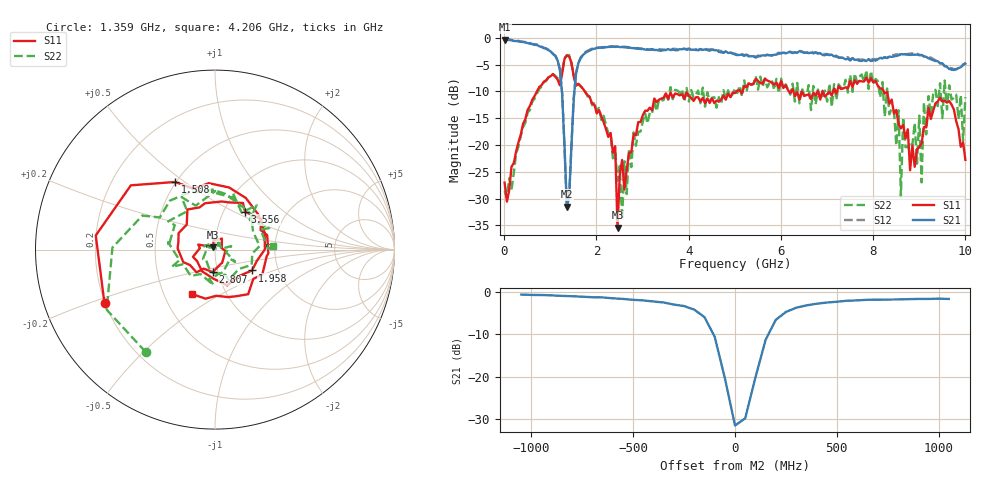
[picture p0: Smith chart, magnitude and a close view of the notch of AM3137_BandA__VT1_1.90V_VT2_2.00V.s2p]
! Date/Time: Tue, Nov 13, 2018 4:48 PM
! Network Analyzer: Agilent Technologies E8364B Rev: A.07.50.67
! Sweep from 0.010 to 10.000 GHz, 201 Points, Sweep Type: LIN
! Power Supply: 1.901 V, -0.000 A
# Hz S DB R 50
!freq MagS11 AngS11 MagS21 AngS21 MagS12 AngS12 MagS22 AngS22
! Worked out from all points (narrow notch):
!   201 points, 10 MHz to 10 GHz, reference 50 ohm
!   highest |S21| = -0.35 dB at 10 MHz (marker M1); lowest = -31.5 dB at 1.359 GHz (marker M2)
!   notch at M2: 28.6 dB deep, 183 MHz wide at half that depth
!   lowest |S11| = -35.4 dB at 2.458 GHz (marker M3), VSWR 1.03, Z = 49 + j1.34 ohm
!   |S11| at or under -10 dB: start of sweep to 710.1 MHz; 1.746 GHz to 5.039 GHz (3.293 GHz wide, 97.1 % of centre); 8.231 GHz to end of sweep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
!   |S22| runs from -34.0 to -3.2 dB; largest |S21 - S12| = 0.03
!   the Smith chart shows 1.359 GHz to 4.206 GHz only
!   S11 on the Smith chart (normalised r, x): 1.359 GHz: 0.20, -0.22; 1.508 GHz: 0.50, +0.46; 1.958 GHz: 1.47, -0.36; 2.807 GHz: 0.94, -0.24; 3.556 GHz: 1.26, +0.57; 4.206 GHz: 0.69, -0.37
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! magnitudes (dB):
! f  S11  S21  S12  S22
! 10 MHz  -27.0  -0.4  -0.3  -28.6
! 1.159 GHz  -7.8  -4.2  -4.1  -7.5
! 1.359 GHz  -3.3  -31.5  -31.4  -3.2
! 1.508 GHz  -7.2  -11.4  -11.3  -7.0
! 1.708 GHz  -9.5  -3.2  -3.2  -9.5
! 1.958 GHz  -12.5  -2.1  -2.0  -12.1
! 2.408 GHz  -20.2  -1.7  -1.6  -21.4
! 2.458 GHz  -35.4  -1.6  -1.7  -26.6
! 2.807 GHz  -18.0  -2.0  -1.9  -17.7
! 3.357 GHz  -11.6  -2.4  -2.2  -11.6
! 3.556 GHz  -11.4  -2.1  -2.3  -11.6
! 4.206 GHz  -11.1  -2.3  -2.3  -9.8
! 5.005 GHz  -10.3  -3.1  -3.0  -9.4
! 6.703 GHz  -10.3  -2.9  -2.8  -9.0
! 8.352 GHz  -12.3  -3.5  -3.5  -14.3
! 8.551 GHz  -16.1  -3.3  -3.1  -13.5
! 8.601 GHz  -16.9  -3.0  -3.1  -29.6
! 8.651 GHz  -16.3  -3.1  -3.2  -14.9
! 9.001 GHz  -20.4  -3.2  -3.2  -14.5
! 9.051 GHz  -19.7  -3.2  -3.2  -27.0
! 9.101 GHz  -16.7  -3.4  -3.5  -12.1
! 10 GHz  -22.8  -4.8  -4.7  -11.1
